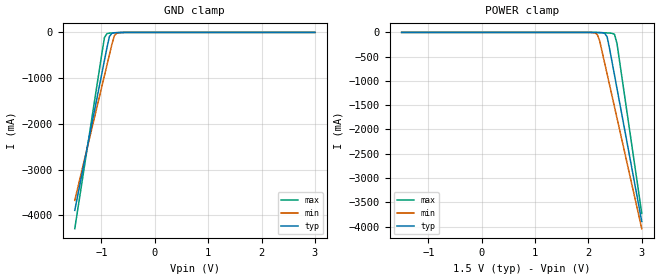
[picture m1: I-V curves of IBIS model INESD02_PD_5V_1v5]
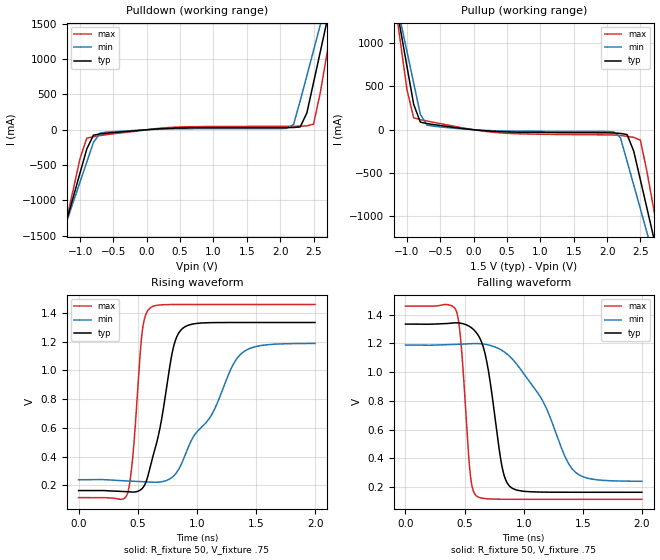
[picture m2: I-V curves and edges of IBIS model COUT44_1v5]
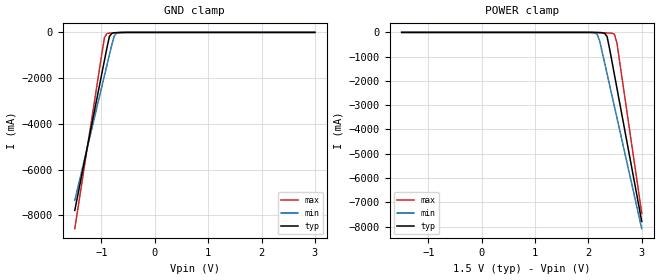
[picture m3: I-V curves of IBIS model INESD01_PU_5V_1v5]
|   This file is an IBIS representation of the   |
|   Integrated Devices Technology , Inc.   |
|   ICS830154I-08   |
|   1:4 Fanout Buffer   |
[IBIS Ver]   4.1
[File name]   830154i_08.ibs
[File Rev]   1.1
| Rev 1.1 June2, 2010
|Added missing 3.3V models.
[Date]   2 Jul 2010
[Source]   Originated at Integrated Device Technology, Inc.
[Disclaimer]
IDT hereby grants the user of this IBIS model a non-exclusive,
nontransferable license to use this IBIS model under the following terms.
Before using this IBIS model, the user should read this license.
If the user does not accept these terms,  the IBIS model should be
returned to IDT within 30 days.
   The user is granted this license only to use the IBIS model and
is not granted rights to sell, load, rent, lease or license the IBIS
model in whole or in part, or in modified form to anyone other than
user. User may modify the IBIS model to suit its specific
applications but rights to derivative works and such modifications
shall belong to IDT.
   This IBIS model is provided on an "AS IS" basis and IDT makes
absolutely no warranty with respect to the information contained
herein. IDT DISCLAIMS AND CUSTOMER WAIVES ALL WARRANTIES, EXPRESS
OR IMPLIED, INCLUDING WARRANTIES OF MERCHANTABILITY OR FITNESS FOR
A PARTICULAR PURPOSE. The entire risk as to quality and performance
is with the Customer. ACCORDINGLY, IN NO EVENT SHALL THE COMPANY BE
LIABLE FOR ANY DAMAGES, WHETHER IN CONTRACT OR TORT,INCLUDING ANY
LOST PROFITS OR OTHER INCIDENTAL, CONSEQUENTIAL, EXEMPLARY, OR
PUNITIVE DAMAGES ARISING OUT OF THE USE OR APPLICATION OF THE IBIS
model provided in this package. Further, IDT reserves the right to
make changes without notice to any product herein to improve
reliability, function, or design. IDT does not convey any license
under patent rights or any other intellectual property rights,
including those of third parties.
   IDT is not obligated to provide maintenance or support
for the licensed IBIS model.
[Copyright]   Copyright 2008 by Integrated Device Technology, Inc.
[Component]   830154GI_08
[Manufacturer] Integrated Device Technology, Inc.
[Package]
|TSSOP 8 Lead
|   typ   min   max
R_pkg   52.5m   48.8m   56.2m
L_pkg   1.381nH   1.275nH   1.486nH
C_pkg   0.236pF   0.230pF   0.242pF
[Pin]   signal_name   model_name   R_pin   L_pin   C_pin
1   CLK_IN   INESD02_PD_5V   56.2m   1.486n   0.242p
2   Q1   COUT44   48.8m   1.275n   0.230p
3   Q2   COUT44   48.8m   1.275n   0.230p
4   Q3   COUT44   56.2m   1.468n   0.242p
5   Q4   COUT44   56.2m   1.486n   0.242p
6   GND   GND   48.8m   1.275n   0.230p
7   VDD   POWER   48.8m   1.275n   0.230p
8   OE   INESD01_PU_5V   56.2m   1.468n   0.242p
[Component]   830154M_08
[Manufacturer] Integrated Device Technology, Inc.
[Package]
|SOIC 8 Lead
|   typ   min   max
R_pkg   57.05m   55.5m   58.6m
L_pkg   1.769nH   1.570nH   1.968nH
C_pkg   0.269pF   0.252pF   0.286pF
[Pin]   signal_name   model_name   R_pin   L_pin   C_pin
1   CLK_IN   INESD02_PD_5V   58.6m   1.968n   0.286p
2   Q1   COUT44   55.5m   1.570n   0.252p
3   Q2   COUT44   55.5m   1.570n   0.252p
4   Q3   COUT44   56.6m   1.968n   0.286p
5   Q4   COUT44   58.6m   1.968n   0.286p
6   GND   GND   55.5m   1.570n   0.252p
7   VDD   POWER   55.5m   1.570n   0.252p
8   OE   INESD01_PU_5V   56.6m   1.968n   0.286p
[Model Selector] INESD02_PD_5V
INESD02_PD_5V_1v5  Buffer selection for 1v5
INESD02_PD_5V_1v8  Buffer selection for 1v8
INESD02_PD_5V_2v5  Buffer selection for 2v5
INESD02_PD_5V_3v3  Buffer selection for 3v3
[Model Selector] COUT44
COUT44_1v5  Buffer selection for 1v5
COUT44_1v8  Buffer selection for 1v8
COUT44_2v5  Buffer selection for 2v5
COUT44_3v3  Buffer selection for 3v3
[Model Selector] INESD01_PU_5V
INESD01_PU_5V_1v5  Buffer selection for 1v5
INESD01_PU_5V_1v8  Buffer selection for 1v8
INESD01_PU_5V_2v5  Buffer selection for 2v5
INESD01_PU_5V_3v3  Buffer selection for 3v3
| Models and submodels in the file (12): INESD02_PD_5V_1v5 (Input), COUT44_1v5 (Output), INESD01_PU_5V_1v5 (Input), INESD02_PD_5V_1v8 (Input), COUT44_1v8 (Output), INESD01_PU_5V_1v8 (Input), INESD02_PD_5V_2v5 (Input), COUT44_2v5 (Output), INESD01_PU_5V_2v5 (Input), INESD02_PD_5V_3v3 (Input), COUT44_3v3 (Output), INESD01_PU_5V_3v3 (Input)
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[Model] INESD02_PD_5V_1v5
Model_type   Input
Polarity   Non-Inverting
Vinl = .525V
Vinh = .975V
|   typ   min   max
C_comp   2pF   1.5pF   2.5pF
|   typ   min   max
[Voltage range]  1.5V   1.425V   1.575V
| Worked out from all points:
|   GND clamp passes 1 mA (typ) near -0.59 V on its own axis
[GND_clamp]
|Voltage   I(typ)   I(min)   I(max)
-1.5V     -3.894A    -3.674A    -4.294A
-989.7mV  -882.2mA   -1.169A    -444.2mA
-943.3mV  -608.7mA   -941.9mA   -111.1mA
-896.9mV  -335.3mA   -714.7mA   -27.01mA
-850.5mV  -87.6mA    -487.5mA   -16.04mA
-804.1mV  -19.87mA   -260.5mA   -12.43mA
-757.7mV  -7.291mA   -70.56mA   -9.686mA
-711.3mV  -3.958mA   -16.84mA   -7.19mA
-664.9mV  -2.373mA   -4.397mA   -4.95mA
3V        58.45uA    73.08uA    45.29uA
[POWER_clamp]
|Voltage   I(typ)   I(min)   I(max)
-1.5V     58.45uA    71.26uA    46.42uA
2.119V    -1.34mA    -9.928mA   -1.015mA
2.165V    -2.373mA   -40.44mA   -2.119mA
2.211V    -3.958mA   -173.5mA   -3.736mA
2.304V    -19.87mA   -627.6mA   -8.12mA
2.351V    -87.6mA    -854.8mA   -10.7mA
2.397V    -335.3mA   -1.082A    -13.62mA
2.49V     -882.2mA   -1.537A    -40.88mA
2.536V    -1.156A    -1.765A    -228.5mA
3V        -3.894A    -4.043A    -3.728A
[Model] COUT44_1v5
Model_type   Output
Polarity   Non-Inverting
Vmeas = .8
Rref = 50
Cref = 0
Vref = .75
|   typ   min   max
C_comp   2pF   1.5pF   2.5pF
|   typ   min   max
[Voltage range]  1.5V   1.425V   1.575V
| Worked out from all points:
|   slope of the pulldown table from 0 to 0.225 V, typ, clamps not added: 15 ohm
|   slope of the pullup table from 0 to 0.225 V, typ, clamps not added: 15.1 ohm
|   rising waveform, R_fixture 50, V_fixture .75: 20-80 % time 159ps typ, 372ps min, 71.5ps max; typ from 0.164 V to 1.33 V
|   falling waveform, R_fixture 50, V_fixture .75: 20-80 % time 124ps typ, 348ps min, 66.3ps max; typ from 1.33 V to 0.164 V
[pulldown]
|Voltage   I (typ)   I (min)   I (max)
-3.3V     -8.323A    -7.168A    -10.22A
-1.3V     -1.614A    -1.572A    -1.688A
-900mV    -271.8mA   -457.1mA   -119.5mA
-700mV    -59.3mA    -46.39mA   -82.97mA
2.1V      30.75mA    19.84mA    48.6mA
2.2V      31.86mA    73.93mA    49.02mA
2.4V      237.7mA    764.4mA    55.05mA
2.5V      666.9mA    1.121A     78.82mA
2.6V      1.097A     1.479A     517.4mA
2.7V      1.529A     1.838A     1.069A
2.8V      1.961A     2.196A     1.622A
6.6V      18.72A     16.1A      23.02A
[pullup]
|Voltage   I (typ)   I (min)   I (max)
-3.3V     10.79A     9.265A     13.29A
-1.2V     1.603A     1.626A     1.578A
-1.1V     1.166A     1.264A     1.019A
-900mV    294.2mA    540.3mA    138.3mA
-700mV    71.14mA    53.15mA    101mA
2.1V      -37.71mA   -24.67mA   -60.94mA
2.3V      -55.71mA   -363.8mA   -76.05mA
2.5V      -580.7mA   -915.6mA   -120.9mA
2.6V      -914.4mA   -1.193A    -492.4mA
2.7V      -1.249A    -1.47A     -919.4mA
2.8V      -1.583A    -1.748A    -1.347A
6.6V      -14.33A    -12.39A    -17.57A
[Ramp]
|   typ   min   max
dV/dt_r   .944/.233n   .853/.277n   1.04/.188n
dV/dt_f   .944/.199n   .853/.245n   1.04/.152n
[Rising Waveform]
R_fixture = 50
V_fixture = .75
V_fixture_max = .7875
V_fixture_min = .7125
C_fixture = 0.0p
| Time   typ   min   max
0s        163.8mV    239.2mV    114.8mV
411.6ps   155.6mV    230.9mV    139.1mV
459.9ps   153.3mV    229.3mV    415.3mV
537.6ps   178.5mV    226.1mV    1.267V
602.7ps   320.2mV    223mV      1.433V
690.9ps   611.4mV    223.8mV    1.456V
800.1ps   1.156V     262.8mV    1.459V
877.8ps   1.291V     364.9mV    1.459V
1.376ns   1.334V     1.116V     1.459V
1.999ns   1.334V     1.188V     1.459V
[Falling Waveform]
R_fixture = 50
V_fixture = .75
V_fixture_max = .7875
V_fixture_min = .7125
C_fixture = 0.0p
| Time   typ   min   max
0s        1.334V     1.188V     1.459V
430.5ps   1.343V     1.193V     1.423V
472.5ps   1.339V     1.194V     1.175V
548.1ps   1.314V     1.198V     287.5mV
600.6ps   1.273V     1.199V     138.1mV
678.3ps   1.109V     1.193V     119.4mV
812.7ps   357.6mV    1.153V     115.3mV
882ps     205.1mV    1.109V     115mV
1.43ns    163.9mV    308.6mV    114.8mV
1.999ns   163.8mV    240.2mV    114.8mV
[Model] INESD01_PU_5V_1v5
Model_type   Input
Polarity   Non-Inverting
Vinl = .525V
Vinh = .975V
|   typ   min   max
C_comp   2pF   1.5pF   2.5pF
|   typ   min   max
[Voltage range]  1.5V   1.425V   1.575V
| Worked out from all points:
|   GND clamp passes 1 mA (typ) near -0.55 V on its own axis
[GND_clamp]
|Voltage   I(typ)   I(min)   I(max)
-1.5V     -7.788A    -7.349A    -8.588A
-989.7mV  -1.764A    -2.339A    -888.5mA
-943.3mV  -1.217A    -1.884A    -222.2mA
-896.9mV  -670.7mA   -1.429A    -54.04mA
-850.5mV  -175.2mA   -975.1mA   -32.1mA
-804.1mV  -39.77mA   -521mA     -24.89mA
-757.7mV  -14.61mA   -141.1mA   -19.4mA
-711.3mV  -7.942mA   -33.7mA    -14.41mA
-664.9mV  -4.769mA   -8.816mA   -9.928mA
3V        29.22uA    38.37uA    21.51uA
[POWER_clamp]
|Voltage   I(typ)   I(min)   I(max)
-1.5V     29.22uA    36.54uA    22.64uA
2.119V    -2.702mA   -19.88mA   -2.051mA
2.165V    -4.769mA   -80.9mA    -4.262mA
2.211V    -7.942mA   -347.1mA   -7.499mA
2.304V    -39.77mA   -1.255A    -16.27mA
2.351V    -175.2mA   -1.71A     -21.43mA
2.397V    -670.7mA   -2.164A    -27.26mA
2.49V     -1.764A    -3.074A    -81.78mA
2.536V    -2.312A    -3.529A    -457mA
3V        -7.788A    -8.086A    -7.456A
